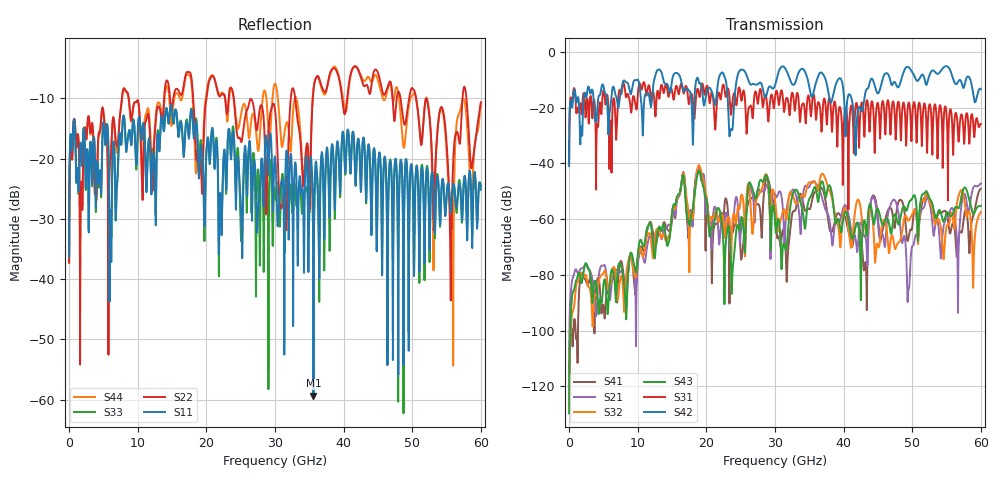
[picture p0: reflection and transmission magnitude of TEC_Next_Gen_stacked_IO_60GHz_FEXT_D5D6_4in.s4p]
!! CHANNEL DESCRIPTION:  Next Generation 28Gbps Press-fit Stacked I/O Connector
!!  with 4" 5-6-5 Megtron 6 Stripline trace on host side and 1.25" 7-5-7 Megtron 6 Microstrip trace on plug side
!! HOST PCB DESCRIPTION:  PCB thickness 3.425 mm
!!  26 Layer Board, 15 GND planes, 4 Layer route-out on Layers 7,11,17,21, 8mil stub on vias
!!  Pairs on following layers
!!  Layer 07 - A02A03 A14A15 D05D06
!!  Layer 11 - D020D3 C05C06 D14D15
!!  Layer 17 - C02C03 B05B06 C14C15
!!  Layer 21 - B02B03 A05A06 B14B15
!! CONNECTOR DESCRIPTION:  Next Generation 28Gbps Press-fit Stacked I/O Connector
!! PLUG-IN CARD DESCRIPTION:  PCB thickness 1mm thick
!!  6 Layer Board, 4 GND planes, 0.35 x 1.4mm mating pads
!!  Micro-strip diff traces referenced to GND plane 3mils down, 2nd GND plane 17mils from top of board
!!  PCB GND planes are symmetric
!! MODEL DESCRIPTION: TE Connectivity S-parameter model produced from Macro-model, Extracted .s4p FEXT (Victim B05B06 - Aggressor D05D06)
!! MODEL DATE: 5/15/2014 CR32f, FPR23
!! MODEL STATUS: Developmental
!! MODEL GEOMETRY: 4 Rows - Rows A, B, C, D. 3 pairs in each row, 12 total pairs
!! MODEL FREQUENCY RANGE: DC to 60 GHz in 10 MHz frequency steps
!! MODEL EDGE RATE LIMITATION: 8.33 ps (Using conservative 0.5/Fmax rule of thumb)
!! TIME-DOMAIN TRANSFORM CAUTIONS:
!! 1.) Do not simulate transient edge rates faster than the number listed above.  Edge
!!  rates faster than this number contain significant spectral content at frequencies
!!  above the model's highest frequency.
!! 2.) Even when simulating edge rates that are slower than the number listed above, be
!!  aware that the best time resolution possible with a direct iFFT is (1 / 2Fmax).
!!  As a result, time resolution is typically not adequate for most time-domain
!!  simulations unless tricks such as frequency-domain zero-padding and windowing are
!!  used to minimize leakage and aliasing.
!! 3.) Because the model has a uniform frequency step, a direct iFFT will result in an
!!  impulse that that has a time length given by either (1 / Fstep) or (1 / 2Fstep),
!!  depending on the transform being used.  Care has been taken in selecting the
!!  frequency step to ensure a settled impulse response for the model.  Therefore,
!!  convolution with the model's impulse response should present no issues.  However,
!!  if directly concatenating s-parameter models in the frequency domain a user must
!!  either interpolate necessary interim frequencies or complete impulse response
!!  zero-padding.  Impulse response zero-padding is more difficult, but more accurate.
!! PORT DEFINITIONS:
!! Port  1  ----->  Host D05		B05 Module <-----  Port  2
!! Port  3  ----->  Host D06		B06 Module <-----  Port  4
! Touchstone data
! Created: 29-Sep-2014 by IdEM R2011 (7.0.3)
# Hz S MA R 50
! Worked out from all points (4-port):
!   6000 points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, 10 MHz to 60 GHz, reference 50 ohm
!   strongest paths, dB at 10 MHz, 15.01 GHz, 30.01 GHz, 45.01 GHz, 60 GHz:
!     S42: -41.0, -10.1, -12.0, -14.9, -13.4
!     S31: -39.6, -14.0, -16.2, -18.5, -25.8
!     S43: -129.7, -57.6, -61.0, -56.4, -55.2
!     S32: -126.9, -57.6, -53.2, -69.4, -57.5
!     S21: -113.6, -59.5, -51.1, -61.8, -47.2
!     S41: -123.4, -60.2, -56.7, -59.7, -49.1
!   lowest |S11| = -59.4 dB at 35.61 GHz (marker M1), VSWR 1.00, Z = 50 - j0.105 ohm
!   |S11| at or under -10 dB: start of sweep to end of sweep
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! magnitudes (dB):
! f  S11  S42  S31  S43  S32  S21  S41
! 10 MHz  -36.3  -41.0  -39.6  -129.7  -126.9  -113.6  -123.4
! 18.84 GHz  -21.4  -10.0  -14.0  -42.8  -40.8  -41.3  -42.8
! 23.82 GHz  -15.8  -27.5  -17.4  -78.5  -61.0  -62.3  -64.9
! 26.34 GHz  -17.2  -11.4  -19.6  -46.8  -51.3  -48.1  -53.0
! 35.61 GHz  -59.4  -14.6  -15.2  -49.3  -46.6  -46.5  -51.3
! 49.45 GHz  -38.0  -5.5  -18.3  -54.7  -60.6  -85.2  -66.9
! 60 GHz  -25.1  -13.4  -25.8  -55.2  -57.5  -47.2  -49.1
